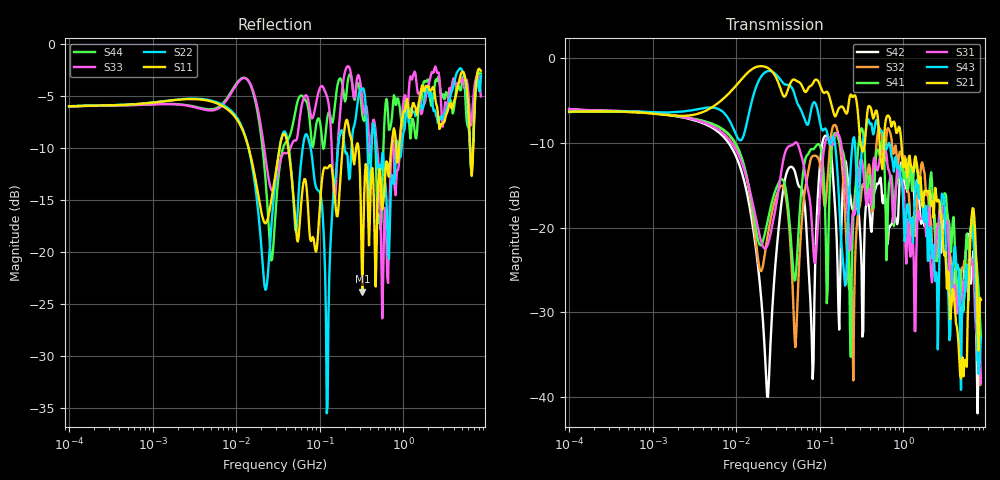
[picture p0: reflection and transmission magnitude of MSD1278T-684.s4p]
# MHz S MA R 50
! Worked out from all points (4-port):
!   498 points, 100 kHz to 8.5 GHz, reference 50 ohm
!   strongest paths, dB at 100 kHz, 1.698 MHz, 29.49 MHz, 500.7 MHz, 8.5 GHz:
!     S21: -6.3, -6.8, -2.2, -7.4, -28.5
!     S43: -6.3, -6.4, -1.9, -8.0, -33.0
!     S31: -6.0, -6.7, -17.8, -13.0, -38.4
!     S41: -6.4, -6.8, -15.6, -10.8, -32.8
!     S32: -6.4, -6.8, -16.6, -8.5, -38.2
!     S42: -6.0, -6.8, -24.3, -14.8, -37.6
!   lowest |S11| = -23.8 dB at 324.4 MHz (marker M1), VSWR 1.14, Z = 56.1 - j3.13 ohm
!   |S11| at or under -10 dB: 41.99 MHz to 187.9 MHz (145.9 MHz wide, 127 % of centre); 291.3 MHz to 720.2 MHz (428.9 MHz wide, 84.8 % of centre); 6.33 GHz to 6.872 GHz (542.9 MHz wide, 8.23 % of centre)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
0.1  0.5028 6.7  0.4819 7.0  0.5008 -8.2  0.4805 -174.6
     0.4819 7.0  0.5035 6.7  0.4804 -174.5  0.4996 -8.4
     0.5008 -8.2  0.4804 -174.5  0.5014 6.7  0.4827 6.9
     0.4805 -174.6  0.4996 -8.4  0.4827 6.9  0.5022 6.9
8.022742  0.4832 -30.6  0.6128 19.9  0.3357 -101.9  0.3577 78.4
          0.6128 19.9  0.4921 -32.0  0.3551 77.6  0.3182 -103.7
          0.3357 -101.9  0.3551 77.6  0.5521 3.5  0.4406 -8.9
          0.3577 78.4  0.3182 -103.7  0.4406 -8.9  0.5619 1.1
23.46849  0.142 -13.9  0.8777 -8.1  0.07768 160.8  0.1065 54.7
          0.8777 -8.1  0.07155 4.5  0.08552 59.5  0.01012 -6.0
          0.07768 160.8  0.08552 59.5  0.2511 -41.3  0.8346 1.3
          0.1065 54.7  0.01012 -6.0  0.8346 1.3  0.1752 -60.4
124.3153  0.2538 -27.9  0.6273 -39.1  0.3418 46.5  0.04282 57.3
          0.6273 -39.1  0.01842 57.9  0.1991 49.5  0.3417 -1.6
          0.3418 46.5  0.1991 49.5  0.5477 -34.9  0.3525 -65.3
          0.04282 57.3  0.3417 -1.6  0.3525 -65.3  0.4519 7.5
324.4107  0.0647 -25.4  0.2812 -58.8  0.2424 -32.9  0.3806 -25.2
          0.2812 -58.8  0.6138 -36.3  0.1782 21.4  0.02275 -104.5
          0.2424 -32.9  0.1782 21.4  0.5286 -76.2  0.3098 1.3
          0.3806 -25.2  0.02275 -104.5  0.3098 1.3  0.4559 -68.6
2652.059  0.4262 126.0  0.1458 21.7  0.1054 113.1  0.08236 107.9
          0.1458 21.7  0.4207 144.4  0.09416 113.0  0.09181 97.0
          0.1054 113.1  0.09416 113.0  0.732 114.6  0.03601 171.4
          0.08236 107.9  0.09181 97.0  0.03601 171.4  0.6991 122.0
8500  0.7457 -51.4  0.0375 -106.1  0.01206 -114.8  0.02282 -131.1
      0.0375 -106.1  0.7059 -39.5  0.0123 -64.2  0.01313 -85.2
      0.01206 -114.8  0.0123 -64.2  0.5614 -50.7  0.0223 1.0
      0.02282 -131.1  0.01313 -85.2  0.0223 1.0  0.7233 -48.9
